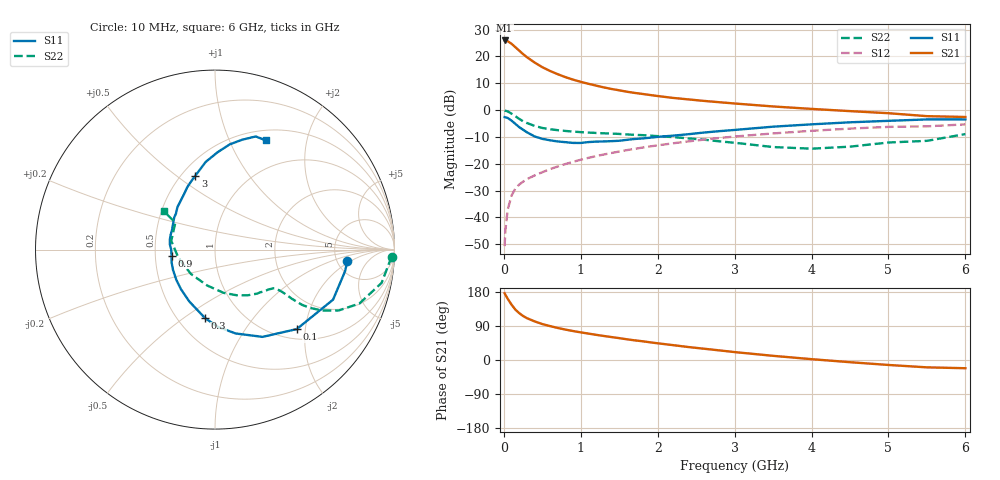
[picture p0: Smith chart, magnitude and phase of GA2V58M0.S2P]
! Infineon Technologies  Discrete & RF Semiconductors
! BF775
! Si NPN RF Bipolar Junction Transistor in SOT23
! VCE = 2.5 V  IC = 8 mA
! Common Emitter S-Parameters:  May  1996
# GHz  S  MA  R  50
!  f  S11  S21  S12  S22
! GHz  MAG  ANG  MAG  ANG  MAG  ANG  MAG  ANG
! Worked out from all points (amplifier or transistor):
!   36 points, 10 MHz to 6 GHz, reference 50 ohm
!   highest |S21| = 26.0 dB at 10 MHz (marker M1)
!   |S21| within 3 dB of that: start of sweep to 169 MHz
!   unconditionally stable (mu >= 1): 621.8 MHz to 3.567 GHz
!   at 250 MHz: K = 0.63, MSG = 23.8 dB, |S12| = -26.7 dB
!   at 1.4 GHz: K = 1.13, MAG = 9.8 dB, |S12| = -16.0 dB
!   at 6 GHz: K = 0.97, MSG = 1.4 dB, |S12| = -5.3 dB
!   S11 on the Smith chart (normalised r, x): 10 MHz: 6.20, -1.74; 100 MHz: 1.21, -1.80; 300 MHz: 0.68, -0.61; 900 MHz: 0.61, -0.04; 3 GHz: 0.58, +0.59; 6 GHz: 0.62, +1.37
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0.01  0.7403 -4.9  19.9 176.2  0.0029 88.4  0.9855 -2.3
0.02  0.7348 -9.4  19.69 172.2  0.0057 83.9  0.9723 -4.6
0.05  0.7144 -23.0  19.28 161.6  0.0139 79.3  0.9467 -11.3
0.1  0.6353 -44.2  17.26 146.1  0.0254 70.3  0.8586 -20.5
0.15  0.5538 -61.4  14.89 132.9  0.0345 64.7  0.7679 -26.2
0.2  0.4811 -76.2  12.87 123.6  0.0409 61.2  0.6855 -29.7
0.25  0.4306 -87.9  11.07 116.2  0.0463 59.6  0.6207 -31.5
0.3  0.3856 -98.3  9.694 110.4  0.0516 59.1  0.5747 -32.4
0.4  0.3227 -116.3  7.717 101.9  0.0604 59.4  0.5074 -32.6
0.5  0.2908 -130.8  6.315 94.8  0.0694 60.2  0.4647 -32.3
0.6  0.2734 -142.1  5.373 89.5  0.0793 60.9  0.4399 -32.2
0.7  0.2601 -154.0  4.676 84.6  0.0887 61.3  0.4223 -32.4
0.9  0.2444 -172.0  3.698 76.4  0.1085 61.8  0.397 -33.0
1.1  0.2533 173.3  3.094 69.7  0.1287 61.5  0.3814 -35.1
1.3  0.2604 161.9  2.651 63.4  0.1487 60.4  0.369 -37.3
1.6  0.279 146.0  2.201 54.6  0.1793 58.3  0.352 -42.0
2.2  0.3335 124.8  1.688 39.2  0.2405 52.9  0.3137 -54.2
3  0.4265 104.8  1.328 20.9  0.3211 43.4  0.246 -78.6
3.5  0.4909 96.1  1.169 11.0  0.3672 37.0  0.2046 -102.4
4.5  0.5922 82.0  0.957 -5.8  0.4519 23.7  0.2081 -166.3
5.5  0.67 70.2  0.771 -19.4  0.4982 9.1  0.2671 145.8
6  0.6709 65.2  0.744 -21.7  0.5417 5.0  0.3574 143.1
